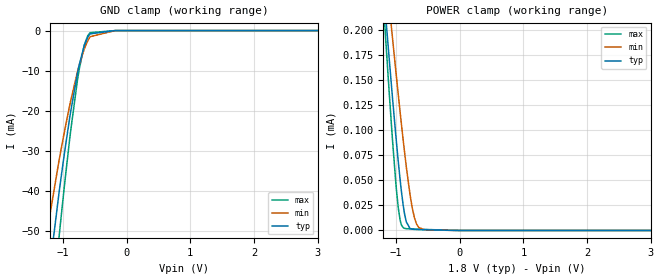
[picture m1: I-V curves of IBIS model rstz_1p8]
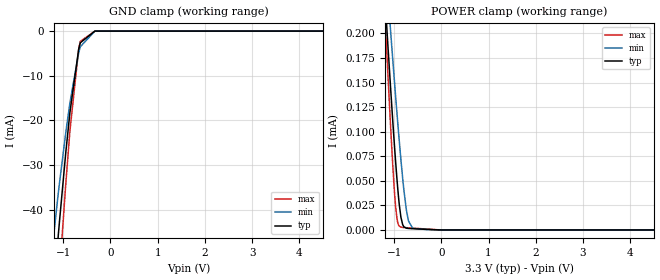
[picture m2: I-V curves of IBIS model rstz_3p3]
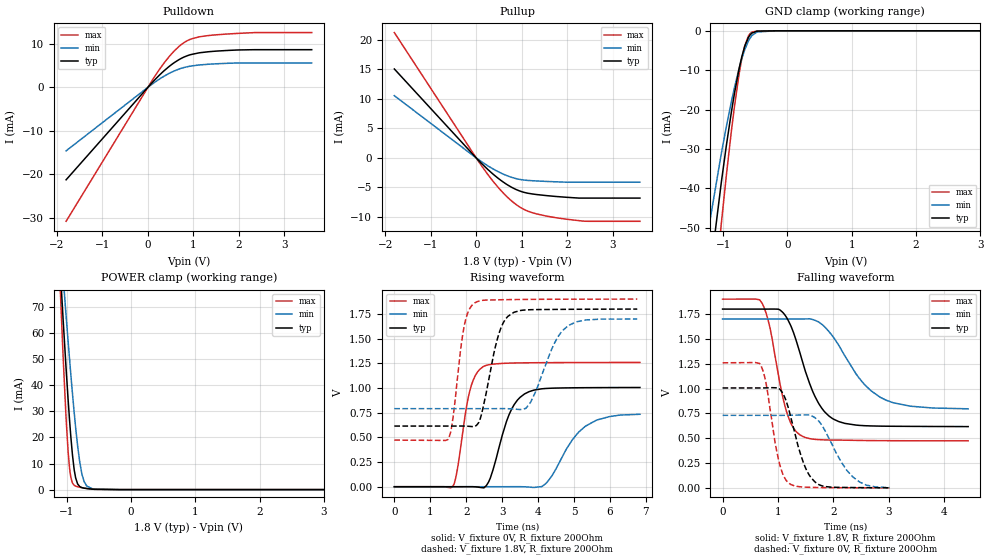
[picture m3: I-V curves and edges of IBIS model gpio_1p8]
|Texas Instruments Incorporated
| OPT3101 ToF based Long Range Proximity and Distance Sensor AFE
| Marketing part#   Digital Voltage Range   Package-type   #pins
| OPT3101   1.7V-3.6V   QFN   28
[IBIS Ver]   4.1
[File name]   opt3101.ibs
[File Rev]   1.0
[Date]   06/18/2018
[Source]
| Texas Instruments Incorporated.
| Analog-eLab Design Center, HPA
| 12500 TI Blvd
| Dallas, TX -75243
[Notes]   Revision History:
| Rev 1.0: 06/18/2018
| - Initial version of the model
| - Model generated from simulations in TISPICE
| - Model matched to SPICE simulation
| - C_comp although listed in numerical order of value are
|   obtained from varying PVT conditions. For PVT conditions for
|   each specific value refer the buffer description under
|   respective [Model]. IBIS model user is responsible for using
|   appropriate C_comp to simulate for Signal Integrity.
|* EXCEPTION:   *
|* - For models i2c_clkdata,There will be a leakage current in the POWER   *
|*   clamp I-V Table because of two resistors(R0 & R1) connected to Pad.*
[Disclaimer]
| This model is designed as an aid for customers of Texas Instruments.
| TI and its licensors and suppliers make no warranties, either expressed
| or implied, with respect to this  model, including the warranties of
| merchantability or fitness for a particular purpose. The model is
| provided solely on an "as is" basis. The entire risk as to its quality
| and performance is with the customer.
[Copyright]
(C) Copyright 2018 Texas Instruments Incorporated.All rights reserved.
|   OPT8320
[Component]   OPT3101
[Manufacturer]   TI
[Package]   |28 QFN package
|   typ   min   max
R_pkg   0.0712   0.0262   0.1046
L_pkg   0.9785nH   0.5979nH   1.4931nH
C_pkg   0.3322pF   0.3071pF   0.4589pF
[Pin]  signal_name   model_name   R_pin   L_pin   C_pin
1   A1   i2c_addr   NA   NA   NA
2   A2   i2c_addr   NA   NA   NA
3   IOVSS   GND   NA   NA   NA
4   TX2   NC   NA   NA   NA
5   TX1   NC   NA   NA   NA
6   VSSL   GND   NA   NA   NA
7   TX0   NC   NA   NA   NA
8   IOVSS   GND NA   NA   NA
9   IOVDD   POWER NA   NA   NA
10   IOVSS   POWER NA   NA   NA
11   GP1   gpio   NA   NA   NA
12   GP2   gpio   NA   NA   NA
13   SCL_S   i2c_clkdata   NA   NA   NA
14   SDA_S   i2c_clkdata   NA   NA   NA
15   SCL_M   i2c_clkdata   NA   NA   NA
16   SDA_M   i2c_clkdata   NA   NA   NA
17   RST_MS   rst_ms_z   NA   NA   NA
18   REG_MODE  rst_ms_z   NA   NA   NA
19   DVDD   POWER   NA   NA   NA
20   AVDD3   POWER   NA   NA   NA
21   AVDD   POWER   NA   NA   NA
22   NC   NC   NA   NA   NA
23   AVSS   GND   NA   NA   NA
24   INM   in_afe   NA   NA   NA
25   INP   in_afe   NA   NA   NA
26   AVSS   GND   NA   NA   NA
27   AVSS   GND   NA   NA   NA
28   A0   i2c_addr   NA   NA   NA
|   Model Selectors
[Model Selector] rst_ms_z
rstz_1p8   1.8V   digital Input
rstz_3p3   3.3V   digital Input
[Model Selector] gpio
gpio_1p8   1.8V   digital IO
gpio_3p3   3.3V   digital IO
[Model Selector] i2c_addr
i2c_addr_1p8  1.8V   digital Input
[Model Selector] i2c_clkdata
i2c_clkdata_1p8   1.8V   digital IO_open_drain
i2c_clkdata_3p3   3.3V   digital IO_open_drain
[Model Selector] in_afe
in_afe_1p8   1.8V   digital Input
| Models and submodels in the file (8): rstz_1p8 (Input), rstz_3p3 (Input), gpio_1p8 (I/O), gpio_3p3 (I/O), i2c_clkdata_1p8 (I/O_open_drain), i2c_clkdata_3p3 (I/O_open_drain), i2c_addr_1p8 (Input), in_afe_1p8 (Input)
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|   rstz_1p8 Model
[Model]   rstz_1p8
Model_type   Input
Vinl = 0.54
Vinh = 1.26
|   typ   min   max
|   (nom PVT)   (fast PVT)   (slow PVT)
C_comp   2.094e-12   1.903e-12   2.287e-12
[Model spec]
|subparameter
Vinl   0.54   0.51   0.57
Vinh   1.26   1.19   1.33
| Where nom  PVT is Nominal Process, 1.8V, 27C
|   Fast PVT is Strong Process,  1.9V, -40C
|   Slow PVT is Weak Process,   1.7V, 125C
[Voltage Range]   1.8   1.7   1.9
|Junction Temperature
[Temperature Range]   27   125   -40
[Power Clamp Reference]   1.8   1.7   1.9
[GND Clamp Reference]   0   0   0
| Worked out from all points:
|   GND clamp passes 1 mA (typ) near -0.58 V on its own axis
[GND Clamp]
|   Voltage   I(typ)   I(min)   I(max)
-1.8V     -235.1mA   -133.1mA   -339.3mA
-1.305V   -71.83mA   -55.34mA   -91.7mA
-1.063V   -40.55mA   -32.52mA   -51.65mA
-1.044V   -38.27mA   -30.86mA   -48.69mA
-973.8mV  -30.2mA    -24.94mA   -38.14mA
-896.4mV  -21.94mA   -18.83mA   -27.26mA
-756mV    -9.362mA   -9.239mA   -10.69mA
-665.7mV  -3.75mA    -4.562mA   -3.604mA
-613.4mV  -1.737mA   -2.608mA   -1.375mA
-572.4mV  -810.3uA   -1.519mA   -523.9uA
-180mV    -497.4nA   -564.7nA   -770.9nA
3.6V      0A         0A         0A
[POWER Clamp]
|   Voltage   I(typ)   I(min)   I(max)
-1.8V     735.1uA    693.3uA    857.7uA
-1.206V   246.5uA    288.5uA    232.3uA
-1.163V   212.5uA    260.1uA    189.5uA
-1.122V   180.7uA    233.3uA    149.7uA
-1.069V   141uA      199.5uA    100.9uA
-964.8mV  67.65uA    134.4uA    21.86uA
-926mV    44.02uA    111.2uA    7.444uA
-874.7mV  19.16uA    81.96uA    2.325uA
-785.1mV  2.297uA    37.3uA     1.574uA
-713.7mV  1.064uA    12.95uA    1.402uA
-550.5mV  726.2nA    684.1nA    1.037uA
3.6V      0A         0A         0A
|   rstz_3p3 Model
[Model]   rstz_3p3
Model_type   Input
Vinl = 0.99
Vinh = 2.31
|   typ   min   max
|   (nom PVT)   (fast PVT)   (slow PVT)
C_comp   2.023e-12   1.832e-12   2.219e-12
[Model spec]
|subparameter
Vinl   0.99   0.90   1.08
Vinh   2.31   2.10   2.52
| Where nom  PVT is Nominal Process, 3.3V, 27C
|   Fast PVT is Strong Process,  3.6V, -40C
|   Slow PVT is Weak Process,   3V, 125C
[Voltage Range]   3.3   3   3.6
|Junction Temperature
[Temperature Range]   27   125   -40
[Power Clamp Reference]   3.3   3   3.6
[GND Clamp Reference]   0   0   0
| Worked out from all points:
|   POWER clamp passes 1 mA (typ) near -2.11 V on its own axis
[GND Clamp]
|   Voltage   I(typ)   I(min)   I(max)
-3.3V     -1.622A    -1.413A    -1.789A
-1.467V   -94.33mA   -71.79mA   -120.1mA
-1.111V   -46.47mA   -36.85mA   -59.33mA
-1.079V   -42.52mA   -33.96mA   -54.21mA
-947.1mV  -27.27mA   -22.78mA   -34.28mA
-858mV    -18.14mA   -15.99mA   -22.25mA
-675mV    -4.21mA    -4.973mA   -4.156mA
-639.6mV  -2.625mA   -3.51mA    -2.314mA
-330mV    -3.16uA    -13.25uA   -3.645uA
6.6V      0A         0A         0A
[POWER Clamp]
|   Voltage   I(typ)   I(min)   I(max)
-3.3V     2.003mA    1.737mA    2.501mA
-1.206V   246.5uA    288.6uA    232.4uA
-1.164V   213.5uA    260.9uA    190.7uA
-1.133V   189.3uA    240.5uA    160.4uA
-1.082V   151uA      208uA      113.1uA
-966.9mV  69.18uA    135.7uA    23.51uA
-920.7mV  41.3uA     108.2uA    7.22uA
-854.7mV  12.85uA    71.23uA    2.892uA
-739.2mV  1.82uA     20.26uA    2.305uA
-693.6mV  1.541uA    9.038uA    2.151uA
-606mV    1.302uA    1.737uA    1.861uA
6.6V      0A         0A         0A
|   gpio_1p8 Model
[Model]   gpio_1p8
Model_type   I/O
Polarity   Non-Inverting
Enable   Active-High
Vinl = 0.54
Vinh = 1.26
Vmeas = 0.9
Vref = 0
Cref = 2pF
Rref = 300
|   typ   min   max
|   (nom PVT)   (fast PVT)   (slow PVT)
C_comp   2.314e-12   2.106e-12   2.515e-12
[Model spec]
|subparameter
Vinl   0.54   0.51   0.57
Vinh   1.26   1.19   1.33
| Where nom  PVT is Nominal Process, 1.8V, 27C
|   Fast PVT is Strong Process,  1.9V, -40C
|   Slow PVT is Weak Process,   1.7V, 125C
[Voltage Range]   1.8   1.7   1.9
|Junction Temperature
[Temperature Range]   27   125   -40
[Pullup Reference]   1.8   1.7   1.9
[Pulldown Reference]   0   0   0
[Power Clamp Reference]   1.8   1.7   1.9
[GND Clamp Reference]   0   0   0
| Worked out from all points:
|   slope of the pulldown table from 0 to 0.27 V, typ, clamps not added: 90.7 ohm
|   slope of the pullup table from 0 to 0.27 V, typ, clamps not added: 131 ohm
|   GND clamp passes 1 mA (typ) near -0.58 V on its own axis
|   POWER clamp passes 1 mA (typ) near -0.78 V on its own axis
|   falling waveform, V_fixture 1.8V, R_fixture 200Ohm: 20-80 % time 451ps typ, 685ps min, 306ps max; typ from 1.8 V to 0.617 V
|   rising waveform, V_fixture 0V, R_fixture 200Ohm: 20-80 % time 523ps typ, 792ps min, 341ps max; typ from 0 V to 1 V
|   rising waveform, V_fixture 1.8V, R_fixture 200Ohm: 20-80 % time 422ps typ, 606ps min, 286ps max; typ from 0.614 V to 1.8 V
|   falling waveform, V_fixture 0V, R_fixture 200Ohm: 20-80 % time 309ps typ, 448ps min, 225ps max; typ from 1.01 V to 0.002 V
[Pulldown]
|   Voltage   I(typ)   I(min)   I(max)
-1.8V     -21.3mA    -14.64mA   -30.86mA
138.6mV   1.594mA    1.077mA    2.336mA
321.6mV   3.491mA    2.343mA    5.13mA
467.8mV   4.81mA     3.206mA    7.084mA
579.6mV   5.682mA    3.765mA    8.38mA
736.5mV   6.676mA    4.382mA    9.863mA
943.6mV   7.528mA    4.886mA    11.09mA
1.147V    7.957mA    5.151mA    11.65mA
1.464V    8.296mA    5.386mA    12.05mA
2.379V    8.654mA    5.601mA    12.6mA
3.6V      8.654mA    5.601mA    12.6mA
[GND Clamp]
|   Voltage   I(typ)   I(min)   I(max)
-1.8V     -229.4mA   -136.4mA   -324.1mA
-1.234V   -65.48mA   -50.91mA   -83.76mA
-1.03V    -38.61mA   -31.28mA   -49.11mA
-872.8mV  -20.69mA   -18.03mA   -25.55mA
-756.2mV  -9.942mA   -9.797mA   -11.38mA
-710.3mV  -6.6mA     -7.091mA   -7.076mA
-663.8mV  -3.897mA   -4.757mA   -3.745mA
-604.9mV  -1.604mA   -2.501mA   -1.231mA
-552.6mV  -571.6uA   -1.205mA   -335.5uA
-474mV    -83.6uA    -300.2uA   -29.97uA
-180mV    0A         -257.9nA   0A
3.6V      0A         0A         0A
[Pullup]
|   Voltage   I(typ)   I(min)   I(max)
-1.8V     15.04mA    10.52mA    21.2mA
127.8mV   -1.011mA   -694.5uA   -1.444mA
340.3mV   -2.541mA   -1.729mA   -3.653mA
510.4mV   -3.613mA   -2.435mA   -5.227mA
682.2mV   -4.533mA   -3.019mA   -6.61mA
863.8mV   -5.298mA   -3.474mA   -7.809mA
1.049V    -5.821mA   -3.744mA   -8.708mA
1.246V    -6.112mA   -3.865mA   -9.296mA
1.563V    -6.39mA    -3.983mA   -9.866mA
1.976V    -6.655mA   -4.105mA   -10.36mA
2.389V    -6.795mA   -4.106mA   -10.71mA
3.6V      -6.795mA   -4.106mA   -10.72mA
[POWER Clamp]
|   Voltage   I(typ)   I(min)   I(max)
-1.8V     411mA      341.7mA    540.9mA
-1.105V   86.59mA    98.07mA    80.06mA
-1.067V   70.27mA    85.51mA    57.79mA
-1.012V   47.3mA     67.39mA    28.39mA
-975.5mV  33.65mA    56.1mA     13.87mA
-935.5mV  20.27mA    44.06mA    4.743mA
-880.3mV  7.155mA    28.72mA    1.602mA
-831mV    2.23mA     16.99mA    1.098mA
-763mV    752.5uA    5.919mA    741.6uA
-688.2mV  401uA      1.367mA    429.5uA
-599.2mV  175.8uA    309.4uA    159uA
3.6V      0A         0A         0A
[Ramp]
R_load = 200
|   typ   min   max
dV/dt_r   0.603657/5.22202e-10   0.438286/7.7537e-10   0.755458/3.39341e-10
dV/dt_f   0.711295/4.52207e-10   0.545564/6.91155e-10   0.856494/3.0524e-10
[Falling Waveform]
V_fixture = 1.8V
V_fixture_min = 1.7V
V_fixture_max = 1.9V
R_fixture = 200Ohm
|   Time   V(typ)   V(min)   V(max)
0s        1.8V       1.7V       1.9V
712ps     1.8V       1.7V       1.86V
858ps     1.8V       1.7V       1.605V
1.152ns   1.718V     1.7V       771.6mV
1.396ns   1.359V     1.7V       533.7mV
1.722ns   861.5mV    1.674V     486.3mV
2.092ns   668.7mV    1.44V      481.3mV
2.51ns    627.9mV    1.074V     477.6mV
2.95ns    621.2mV    883mV      475.5mV
4.43ns    617.3mV    796.2mV    473.8mV
[Rising Waveform]
V_fixture = 0V
V_fixture_min = 0V
V_fixture_max = 0V
R_fixture = 200Ohm
|   Time   V(typ)   V(min)   V(max)
0s        1.016nV    46.74nV    574.5pV
1.654ns   -3.413uV   -7.315uV   20.4mV
2.098ns   427.4uV    -11.8uV    968.1mV
2.492ns   -11.55mV   -16.66uV   1.22V
2.672ns   89.04mV    -19.16uV   1.238V
3.194ns   731.1mV    148.2uV    1.252V
3.624ns   940.3mV    -780.4uV   1.255V
4.216ns   995.1mV    32.27mV    1.257V
5.316ns   1.003V     612.7mV    1.258V
6.834ns   1.005V     733.8mV    1.259V
[Rising Waveform]
V_fixture = 1.8V
V_fixture_min = 1.7V
V_fixture_max = 1.9V
R_fixture = 200Ohm
|   Time   V(typ)   V(min)   V(max)
0s        614.5mV    790.7mV    472.3mV
1.494ns   614.5mV    790.7mV    478.9mV
1.614ns   614.5mV    790.7mV    650.7mV
1.95ns    614.2mV    790.7mV    1.638V
2.242ns   610.9mV    790.7mV    1.863V
2.91ns    1.551V     791mV      1.893V
3.158ns   1.725V     790.4mV    1.895V
3.786ns   1.793V     851.6mV    1.898V
4.84ns    1.797V     1.633V     1.899V
6.76ns    1.799V     1.699V     1.9V
[Falling Waveform]
V_fixture = 0V
V_fixture_min = 0V
V_fixture_max = 0V
R_fixture = 200Ohm
|   Time   V(typ)   V(min)   V(max)
0s        1.006V     730.5mV    1.259V
698ps     1.006V     730.4mV    1.224V
794ps     1.007V     730.3mV    1.024V
1.01ns    1.005V     730.2mV    283.9mV
1.108ns   928.3mV    730.5mV    113mV
1.198ns   783.1mV    731.1mV    46.64mV
1.468ns   239.7mV    734.7mV    8.638mV
1.706ns   42.82mV    689.2mV    4.175mV
2.342ns   3.746mV    114.3mV    1.568mV
3.01ns    1.504mV    3.202mV    622uV
